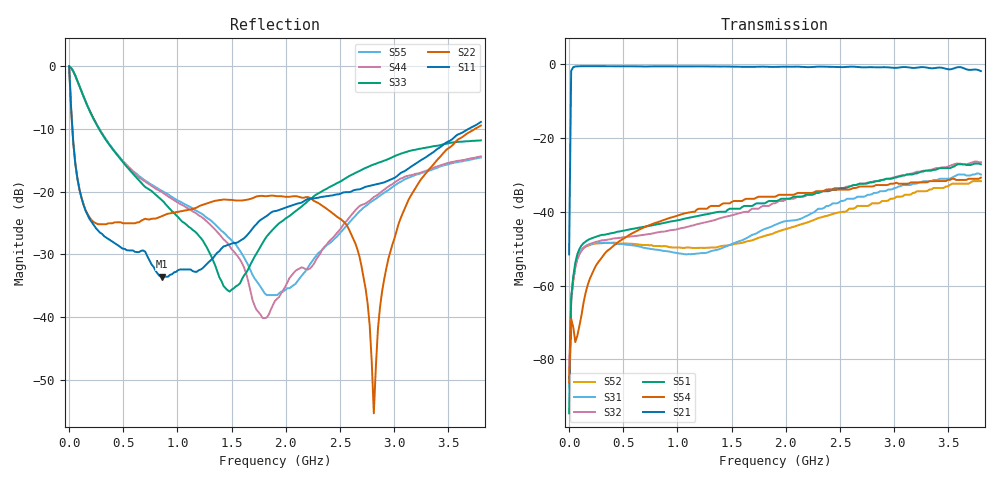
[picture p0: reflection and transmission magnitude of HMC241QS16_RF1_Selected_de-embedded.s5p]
! Hittite Microwave Corporation
! 20 Alpha Road
! Chelmsford, MA 01824
! Tel: 978-250-3343
! Fax: 978-250-3373
! Device: HMC241QS16, DC-3.5 GHz GaAs MMIC SP4T Non-Reflective Switch in 16 lead QSOP package
! Misc: Data was de-embedded to package pins.
!  Port 1 = RFC
!  Port 2 = RF1
!  Port 3 = RF2
!  Port 4 = RF3
!  Port 5 = RF4
!  Vdd  = + 5 V
!  RF1 selected, Vctl= 0/+5 V
!  Data reformated to new Touchstone file format - Tue Jan 09 09:58:23 2007
# MHz S DB R 50
! 5 Port Network Data
! freq  dbS11  angS11  dbS12  angS12  dbS13  angS13  dbS14  angS14
!  dbS15  angS15
!  dbS21  angS21  dbS22  angS22  dbS23  angS23
!  dbS24  angS24  dbS25  angS25
!  dbS31  angS31  dbS32  angS32
!  dbS33  angS33  dbS34  angS34  dbS35  angS35
!  dbS41  angS41
!  dbS42  angS42  dbS43  angS43  dbS44  angS44  dbS45  angS45
!  dbS51  angS51  dbS52  angS52  dbS53  angS53  dbS54  angS54
!  dbS55  angS55
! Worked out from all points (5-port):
!   201 points, 30 kHz to 3.8 GHz, reference 50 ohm
!   strongest paths, dB at 30 kHz, 950 MHz, 1.9 GHz, 2.85 GHz, 3.8 GHz:
!     S21: -51.6, -0.6, -0.7, -0.9, -1.9
!     S54: -86.2, -41.5, -35.9, -32.8, -30.8
!     S51: -94.6, -42.6, -37.1, -31.7, -27.1
!     S32: -84.4, -45.0, -37.7, -31.6, -26.6
!     S31: -87.6, -51.0, -43.6, -34.8, -29.9
!     S52: -84.7, -49.7, -45.7, -37.7, -31.7
!   lowest |S11| = -33.6 dB at 855 MHz (marker M1), VSWR 1.04, Z = 52.1 - j0.0119 ohm
!   |S11| at or under -10 dB: 30.27 MHz to 3.686 GHz (3.656 GHz wide, 197 % of centre)
